FUNCTION_BLOCK DownTyp
VAR_INPUT
END_VAR
VAR_OUTPUT
END_VAR

// NETWORK 1
// instruction list
LD      TRUE
S       deviceDown
R       deviceUp

// NETWORK 2
// instruction list
LD      T#2s
ST      timerDown.PT

// NETWORK 3
// instruction list
LD      TRUE
S       timerDown.IN
CAL     timerDown

END_FUNCTION_BLOCK
